(* Logix 5000 AddOnInstructionDefinition export AMCI_NXFE2_Preset_Encoder_Position; software revision 20.03 *)

ADD_ON_INSTRUCTION AMCI_NXFE2_Preset_Encoder_Position   (* revision 1.0, vendor AMCI *)
VAR_INPUT
   Target_Position : DINT; {required}
END_VAR
VAR_IN_OUT
   NXFE2_output_data : _000A:NXFE2_0986AEB4:O:0; {required}
END_VAR
VAR
   command_data_block : INT[10];
        [0]   // Command Bits MSW
        [1]   // Command Bits LSW
        [2]   // Upper Target Position
        [3]   // Lower Target Position
        [4]   // Upper Programmed Speed
        [5]   // Lower Programmed Speed
END_VAR

ROUTINE Logic   (* ladder *)
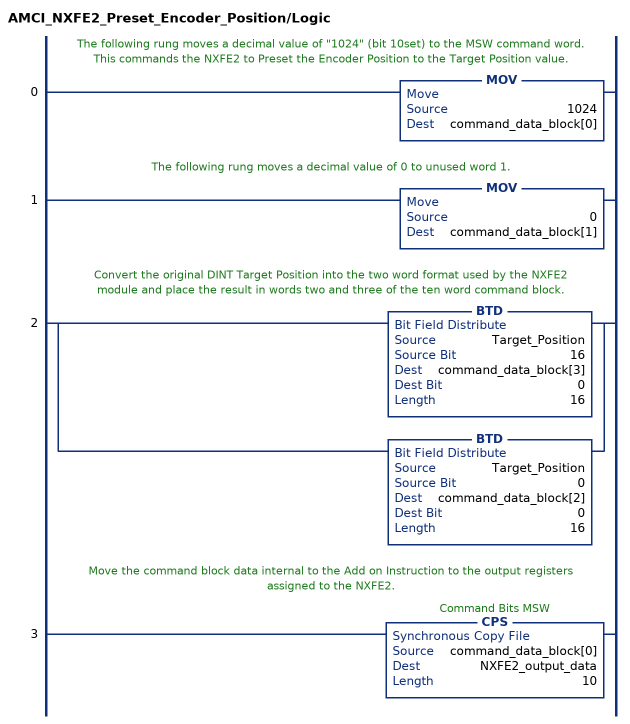
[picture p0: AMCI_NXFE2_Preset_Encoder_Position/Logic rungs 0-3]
   // The following rung moves a decimal value of "1024" (bit 10set) to the MSW command word.  This commands the NXFE2 to Preset the Encoder Position to the Target Position value.
   0: MOV(1024,command_data_block[0]);
   // The following rung moves a decimal value of 0 to unused word 1.
   1: MOV(0,command_data_block[1]);
   // Convert the original DINT Target Position into the two word format used by the NXFE2 module and place the result in words two and three of the ten word command block.
   2: [BTD(Target_Position,16,command_data_block[3],0,16) ,BTD(Target_Position,0,command_data_block[2],0,16) ];
   // Move the command block data internal to the Add on Instruction to the output registers assigned to the NXFE2.
   3: CPS(command_data_block[0],NXFE2_output_data,10);
END_ROUTINE
END_ADD_ON_INSTRUCTION
